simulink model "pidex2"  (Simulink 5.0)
settings: Solver=ode45  StartTime=0.0  StopTime=2  MaxStep=1e-4

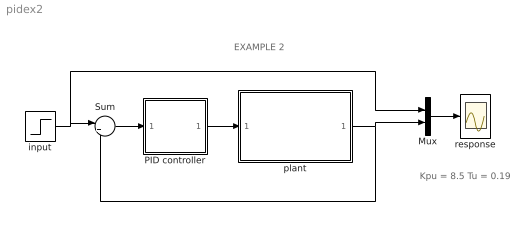
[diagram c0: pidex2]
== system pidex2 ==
  note: EXAMPLE 2
  note: Kpu = 8.5 Tu = 0.19
  Mux : Mux  Inputs=2
  PID controller : Subsystem  mask{Kp=5.1, Ki=53.7, Kd=0.11, sat=2}
      mask prompts: Kp "Proportional gain (Kp)"; Ki "Integral gain (Ki)"; Kd "Derivative gain (Kd)"; sat "Saturation limit [pu]"
      mask help: Proportional-Integral Speed Controller
  Sum : Sum  Inputs=|+-
  input : Step  Time=.05  SampleTime=0
  plant : Subsystem  mask{Ka=1, Ta=0.25, Td=0.05}
      mask prompts: Ka "Gain"; Ta "Time constant [s]"; Td "Time delay [s]"
  response : Scope
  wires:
  plant/1(Out1) -> Sum/2, Mux/2
  Sum/1 -> PID controller/1(er)
  PID controller/1(c) -> plant/1(In1)
  input/1 -> Sum/1, Mux/1
  Mux/1 -> response/1

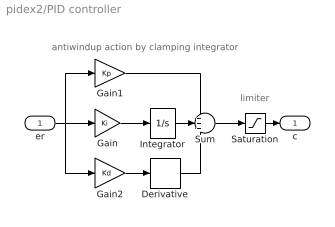
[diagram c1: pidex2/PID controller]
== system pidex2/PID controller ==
  note: antiwindup action by clamping integrator
  note: limiter
  er : Inport
  Derivative : Derivative
  Gain : Gain  Gain=Ki
  Gain1 : Gain  Gain=Kp
  Gain2 : Gain  Gain=Kd
  Integrator : Integrator  LimitOutput=on  UpperSaturationLimit=sat  LowerSaturationLimit=-sat
  Saturation : Saturate  UpperLimit=sat  LowerLimit=-sat
  Sum : Sum  Inputs=+++
  c : Outport  InitialOutput=0
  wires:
  Gain1/1 -> Sum/1
  Gain/1 -> Integrator/1
  er/1 -> Gain/1, Gain1/1, Gain2/1
  Sum/1 -> Saturation/1
  Saturation/1 -> c/1
  Integrator/1 -> Sum/2
  Gain2/1 -> Derivative/1
  Derivative/1 -> Sum/3

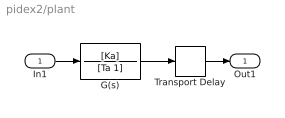
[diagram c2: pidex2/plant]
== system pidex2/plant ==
  In1 : Inport
  G(s) : TransferFcn  Numerator=[Ka]  Denominator=[Ta 1]
  Transport Delay : TransportDelay  DelayTime=Td  BufferSize=2048
  Out1 : Outport
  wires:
  G(s)/1 -> Transport Delay/1
  In1/1 -> G(s)/1
  Transport Delay/1 -> Out1/1
